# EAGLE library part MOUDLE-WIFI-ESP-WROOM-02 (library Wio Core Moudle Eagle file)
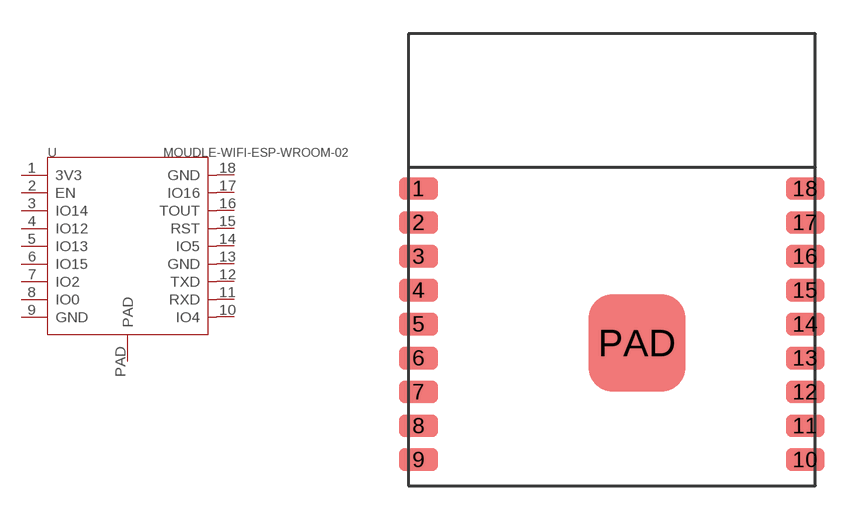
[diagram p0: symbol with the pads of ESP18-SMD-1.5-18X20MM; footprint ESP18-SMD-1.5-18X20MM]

Designator prefix U

## MOUDLE-WIFI-ESP-WROOM-02  [ESP18-SMD-1.5-18X20MM]
1  3V3
2  EN
3  IO14
4  IO12
5  IO13
6  IO15
7  IO2
8  IO0
9  GND
10  IO4
11  RXD
12  TXD
13  GND
14  IO5
15  RST
16  TOUT
17  IO16
18  GND
PAD  PAD

## Footprint ESP18-SMD-1.5-18X20MM (pad centres in mm)
smd 1.7 x 1: 1 0.45,13.15; 2 0.45,11.65; 3 0.45,10.15; 4 0.45,8.65; 5 0.45,7.15; 6 0.45,5.65; 7 0.45,4.15; 8 0.45,2.65; 9 0.45,1.15; 10 17.55,1.15; 11 17.55,2.65; 12 17.55,4.15; 13 17.55,5.65; 14 17.55,7.15; 15 17.55,8.65; 16 17.55,10.15; 17 17.55,11.65; 18 17.55,13.15
smd 4.3 x 4.3: PAD 10.12,6.32

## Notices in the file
http://creativecommons.org/licenses/by-sa/4.0/'
CC-BY-SA
